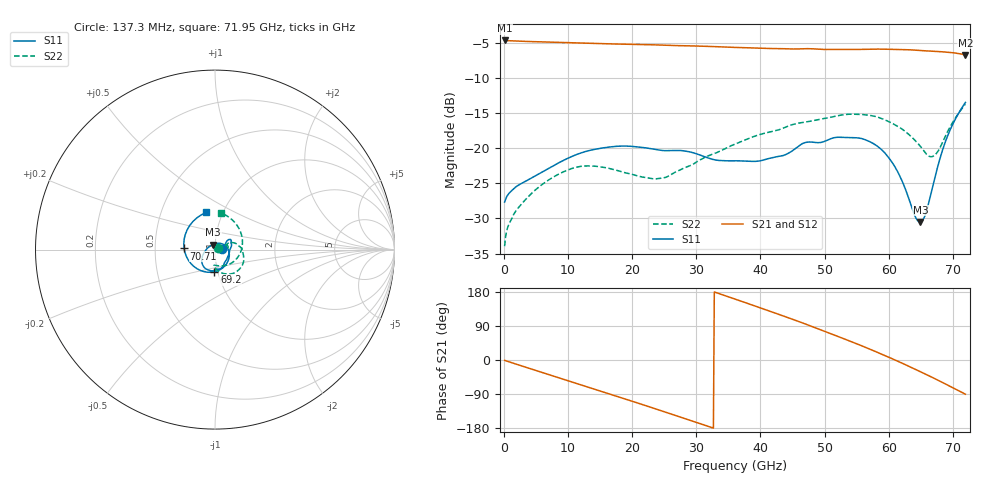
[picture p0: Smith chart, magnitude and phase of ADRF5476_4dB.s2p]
! Device:  ADRF5476
! Description: Flip-Chip, Silicon Digital Step Attenuator
! Frequency:  0.1 GHz -  72 GHz
! Ports:
!  RFC = ATTIN
!  RF1 = ATTOUT
! VDD  =  +3.3 Volts
! VSS  =  -3.3 Volts
! State
! 4dB Attenuation State: D0 = +3.3V, D1 = 0V
! Data:  Data was collected using a calibrated network analyzer
!  The reference plane is the package boundry of ADRF5476 switch.
! Notes: Analog Devices supplies this data as a sample of measured data
!  for this product.  Your particular data for this product may vary.
!  Analog Devices reserves the right to change this data at anytime.
# GHZ  S  DB  R  50
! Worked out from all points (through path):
!   524 points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, 137.3 MHz to 71.95 GHz, reference 50 ohm
!   highest |S21| = -4.61 dB at 137.3 MHz (marker M1); lowest = -6.7 dB at 71.95 GHz (marker M2)
!   group delay of S21, straight-line fit = 16.9 ps
!   lowest |S11| = -30.5 dB at 64.95 GHz (marker M3), VSWR 1.06, Z = 48.9 + j2.76 ohm
!   |S11| at or under -10 dB: start of sweep to end of sweep
!   |S22| runs from -33.9 to -13.7 dB; largest |S21 - S12| = 0.069
!   S11 on the Smith chart (normalised r, x): 137.3 MHz: 1.09, +0.01; 69.2 GHz: 0.96, -0.24; 70.71 GHz: 0.71, +0.01; 71.95 GHz: 0.83, +0.36
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0.1373092  -27.66 7.8  -4.61 -0.9  -4.61 -0.9  -33.95 18.5
1.64771  -25.68 15.3  -4.68 -9.4  -4.68 -9.3  -29.27 20.9
4.256584  -24.26 25.1  -4.77 -23.6  -4.76 -23.6  -26.49 27.1
12.22052  -20.60 36.2  -4.99 -66.5  -4.98 -66.5  -22.55 14.6
18.12481  -19.68 31.7  -5.13 -98.6  -5.13 -98.6  -23.27 5.1
24.16641  -20.23 24.4  -5.26 -131.8  -5.25 -131.8  -24.30 15.0
30.34532  -20.87 8.7  -5.42 -166.4  -5.41 -166.4  -21.76 25.8
36.11231  -21.78 -11.8  -5.60 160.4  -5.60 160.4  -19.37 21.1
42.56584  -21.19 -47.7  -5.76 122.2  -5.76 122.1  -17.43 8.4
48.05821  -19.11 -80.8  -5.79 88.1  -5.79 88.1  -16.07 -7.2
51.90286  -18.42 -98.6  -5.89 63.4  -5.88 63.3  -15.37 -19.8
55.61021  -18.57 -117.7  -5.88 38.7  -5.88 38.7  -15.16 -37.3
60.0041  -21.34 -147.3  -5.87 7.3  -5.86 7.2  -16.18 -61.3
64.12338  -29.70 141.1  -5.99 -24.5  -5.98 -24.5  -18.89 -84.6
64.94723  -30.50 109.5  -6.04 -31.0  -6.04 -31.1  -19.72 -89.5
65.77109  -29.28 78.4  -6.09 -37.5  -6.08 -37.6  -20.72 -94.2
67.00687  -24.84 28.0  -6.16 -47.7  -6.16 -47.1  -21.07 -86.3
68.24265  -20.67 -33.7  -6.22 -58.1  -6.22 -56.0  -19.44 -55.6
69.20382  -18.16 -91.3  -6.28 -66.4  -6.28 -62.7  -17.56 -20.5
69.89036  -16.72 -132.6  -6.34 -72.4  -6.34 -67.4  -16.42 4.8
70.71422  -15.27 177.8  -6.45 -79.5  -6.45 -73.1  -15.22 35.1
71.95  -13.45 103.4  -6.67 -90.2  -6.67 -81.7  -13.69 80.6
